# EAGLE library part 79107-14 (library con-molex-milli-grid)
RECEPTACAL
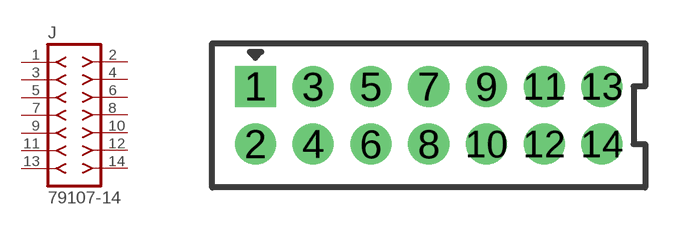
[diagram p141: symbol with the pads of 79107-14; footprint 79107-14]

Designator prefix J

## 79107-14  [79107-14]
1  1  pas
2  2  pas
3  3  pas
4  4  pas
5  5  pas
6  6  pas
7  7  pas
8  8  pas
9  9  pas
10  10  pas
11  11  pas
12  12  pas
13  13  pas
14  14  pas

## Footprint 79107-14 (pad centres in mm)
RECEPTACAL Dual Row, Vertical, Through-Hole
drill 0.914 square: 1 -6,1
drill 0.914: 2 -6,-1; 3 -4,1; 4 -4,-1; 5 -2,1; 6 -2,-1; 7 0,1; 8 0,-1; 9 2,1; 10 2,-1; 11 4,1; 12 4,-1; 13 6,1; 14 6,-1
